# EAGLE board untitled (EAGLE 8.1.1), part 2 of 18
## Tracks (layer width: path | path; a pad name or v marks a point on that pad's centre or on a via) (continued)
S$1112
  Bottom 0: 321.52,97.17 320.59,96.24
S$1113
  Bottom 0: 320.59,96.24 320.33,96.22
S$1114
  Bottom 0: 320.33,96.22 320.22,96.19
S$1115
  Bottom 0: 320.22,96.19 319.92,96.25
S$1116
  Bottom 0: 319.92,96.25 319.57,96.22
S$1117
  Bottom 0: 319.57,96.22 319.24,96.12
S$1118
  Bottom 0: 319.24,96.12 318.94,95.93
S$1119
  Bottom 0: 318.94,95.93 318.7,95.68
S$1120
  Bottom 0: 318.7,95.68 318.53,95.37
S$1121
  Bottom 0: 318.53,95.37 318.44,95.03
S$1122
  Bottom 0: 318.44,95.03 318.44,94.68
S$1123
  Bottom 0: 318.44,94.68 318.53,94.34
S$1124
  Bottom 0: 318.53,94.34 318.7,94.03
S$1125
  Bottom 0: 318.7,94.03 318.94,93.78
S$1126
  Bottom 0: 318.94,93.78 319.24,93.59
S$1127
  Bottom 0: 319.24,93.59 319.57,93.48
S$1128
  Bottom 0: 319.57,93.48 319.92,93.46
S$1129
  Bottom 0: 319.92,93.46 320.22,93.52
S$1130
  Bottom 0: 320.22,93.52 320.33,93.48
S$1131
  Bottom 0: 320.33,93.48 320.68,93.46
S$1132
  Bottom 0: 320.68,93.46 321.03,93.52
S$1133
  Bottom 0: 321.03,93.52 321.34,93.67
S$1134
  Bottom 0: 321.34,93.67 321.61,93.9
S$1135
  Bottom 0: 321.61,93.9 321.82,94.18
S$1136
  Bottom 0: 321.82,94.18 321.94,94.51
S$1137
  Bottom 0: 321.94,94.51 321.99,94.85
S$1138
  Bottom 0: 321.99,94.85 321.94,95.2
S$1139
  Bottom 0: 321.94,95.2 321.82,95.52
S$1140
  Bottom 0: 321.82,95.52 321.61,95.81
S$1141
  Bottom 0: 321.61,95.81 321.5,95.9
S$1142
  Bottom 0: 321.5,95.9 322.27,96.68
S$1143
  Bottom 0: 322.27,96.68 322.32,96.73
S$1144
  Bottom 0: 322.32,96.73 322.35,96.79
S$1145
  Bottom 0: 322.35,96.79 322.38,96.85
S$1146
  Bottom 0: 322.38,96.85 322.4,96.92
S$1147
  Bottom 0: 322.4,96.92 322.4,96.99
S$1148
  Bottom 0: 322.4,96.99 322.4,116.07
S$1149
  Bottom 0: 322.4,116.07 323.2,116.07
S$1150
  Bottom 0: 323.2,116.07 323.28,116.08
S$1151
  Bottom 0: 323.28,116.08 323.35,116.12
S$1152
  Bottom 0: 323.35,116.12 323.41,116.18
S$1153
  Bottom 0: 323.41,116.18 323.45,116.25
S$1154
  Bottom 0: 323.45,116.25 323.46,116.33
S$1155
  Bottom 0: 323.46,116.33 323.46,144.15
S$1156
  Bottom 0: 323.46,144.15 323.45,144.22
S$1157
  Bottom 0: 323.45,144.22 323.41,144.3
S$1158
  Bottom 0: 323.41,144.3 323.35,144.35
S$1159
  Bottom 0: 323.35,144.35 323.28,144.39
S$1160
  Bottom 0: 323.28,144.39 323.2,144.4
S$1161
  Bottom 0: 323.2,144.4 322.4,144.4
S$1162
  Bottom 0: 322.4,144.4 322.4,150.63
S$1163
  Bottom 0: 322.4,150.63 322.4,150.71
S$1164
  Bottom 0: 322.4,150.71 322.38,150.77
S$1165
  Bottom 0: 322.38,150.77 322.35,150.84
S$1166
  Bottom 0: 322.35,150.84 322.32,150.9
S$1167
  Bottom 0: 322.32,150.9 322.27,150.95
S$1168
  Bottom 0: 322.27,150.95 321.84,151.38
S$1169
  Bottom 0: 321.84,151.38 321.95,151.66
S$1170
  Bottom 0: 321.95,151.66 322,152
S$1171
  Bottom 0: 322,152 321.95,152.35
S$1172
  Bottom 0: 321.95,152.35 321.82,152.67
S$1173
  Bottom 0: 321.82,152.67 321.62,152.96
S$1174
  Bottom 0: 321.62,152.96 321.35,153.18
S$1175
  Bottom 0: 321.35,153.18 321.03,153.34
S$1176
  Bottom 0: 321.03,153.34 320.69,153.39
S$1177
  Bottom 0: 320.69,153.39 320.33,153.38
S$1178
  Bottom 0: 320.33,153.38 320.23,153.34
S$1179
  Bottom 0: 320.23,153.34 319.92,153.39
S$1180
  Bottom 0: 319.92,153.39 319.68,153.38
S$1181
  Bottom 0: 319.68,153.38 322.49,156.19
S$1182
  Bottom 0: 322.49,156.19 322.53,156.25
S$1183
  Bottom 0: 322.53,156.25 322.57,156.31
S$1184
  Bottom 0: 322.57,156.31 322.6,156.37
S$1185
  Bottom 0: 322.6,156.37 322.61,156.43
S$1186
  Bottom 0: 322.61,156.43 322.62,156.5
S$1187
  Bottom 0: 322.62,156.5 322.62,171.62
S$1188
  Bottom 0: 322.62,171.62 322.61,171.69
S$1189
  Bottom 0: 322.61,171.69 322.6,171.76
S$1190
  Bottom 0: 322.6,171.76 322.57,171.82
S$1191
  Bottom 0: 322.57,171.82 322.53,171.88
S$1192
  Bottom 0: 322.53,171.88 322.49,171.94
S$1193
  Bottom 0: 322.49,171.94 318.05,176.38
S$1194
  Bottom 0: 318.05,176.38 318.06,176.42
S$1195
  Bottom 0: 318.06,176.42 318.01,176.67
S$1196
  Bottom 0: 318.01,176.67 317.88,176.89
S$1197
  Bottom 0: 317.88,176.89 317.68,177.04
S$1198
  Bottom 0: 317.68,177.04 317.43,177.1
S$1199
  Bottom 0: 317.43,177.1 317.19,177.08
S$1200
  Bottom 0: 317.19,177.08 317.06,177.02
S$1201
  Bottom 0: 317.06,177.02 317.65,177.61
S$1202
  Bottom 0: 317.65,177.61 317.9,177.54
S$1203
  Bottom 0: 317.9,177.54 318.22,177.54
S$1204
  Bottom 0: 318.22,177.54 318.53,177.63
S$1205
  Bottom 0: 318.53,177.63 318.81,177.81
S$1206
  Bottom 0: 318.81,177.81 319.02,178.05
S$1207
  Bottom 0: 319.02,178.05 319.16,178.35
S$1208
  Bottom 0: 319.16,178.35 319.2,178.67
S$1209
  Bottom 0: 319.2,178.67 319.16,178.99
S$1210
  Bottom 0: 319.16,178.99 319.02,179.29
S$1211
  Bottom 0: 319.02,179.29 318.81,179.54
S$1212
  Bottom 0: 318.81,179.54 318.53,179.72
S$1213
  Bottom 0: 318.53,179.72 318.22,179.81
S$1214
  Bottom 0: 318.22,179.81 317.9,179.81
S$1215
  Bottom 0: 317.9,179.81 317.68,179.74
S$1216
  Bottom 0: 317.68,179.74 316.95,180.46
S$1217
  Bottom 0: 316.95,180.46 316.89,180.52
S$1218
  Bottom 0: 316.89,180.52 316.81,180.57
S$1219
  Bottom 0: 316.81,180.57 316.73,180.6
S$1220
  Bottom 0: 316.73,180.6 316.64,180.62
S$1221
  Bottom 0: 316.64,180.62 316.56,180.63
S$1222
  Bottom 0: 316.56,180.63 300.39,180.63
S$1223
  Bottom 0: 300.39,180.63 300.3,180.62
S$1224
  Bottom 0: 300.3,180.62 300.21,180.6
S$1225
  Bottom 0: 300.21,180.6 300.13,180.57
S$1226
  Bottom 0: 300.13,180.57 300.06,180.52
S$1227
  Bottom 0: 300.06,180.52 299.99,180.46
S$1228
  Bottom 0: 299.99,180.46 299.29,179.77
S$1229
  Bottom 0: 299.29,179.77 299.17,179.81
S$1230
  Bottom 0: 299.17,179.81 298.84,179.81
S$1231
  Bottom 0: 298.84,179.81 298.63,179.74
S$1232
  Bottom 0: 298.63,179.74 297.9,180.46
S$1233
  Bottom 0: 297.9,180.46 297.84,180.52
S$1234
  Bottom 0: 297.84,180.52 297.76,180.57
S$1235
  Bottom 0: 297.76,180.57 297.68,180.6
S$1236
  Bottom 0: 297.68,180.6 297.6,180.62
S$1237
  Bottom 0: 297.6,180.62 297.5,180.63
S$1238
  Bottom 0: 297.5,180.63 288.83,180.63
S$1239
  Bottom 0: 288.83,180.63 288.74,180.62
S$1240
  Bottom 0: 288.74,180.62 288.66,180.6
S$1241
  Bottom 0: 288.66,180.6 288.57,180.57
S$1242
  Bottom 0: 288.57,180.57 288.5,180.52
S$1243
  Bottom 0: 288.5,180.52 288.43,180.46
S$1244
  Bottom 0: 288.43,180.46 283.51,175.54
S$1245
  Bottom 0: 283.51,175.54 283.45,175.47
S$1246
  Bottom 0: 283.45,175.47 283.4,175.4
S$1247
  Bottom 0: 283.4,175.4 283.37,175.32
S$1248
  Bottom 0: 283.37,175.32 283.35,175.23
S$1249
  Bottom 0: 283.35,175.23 283.34,175.14
S$1250
  Bottom 0: 283.34,175.14 283.34,173.77
S$1251
  Bottom 0: 283.34,173.77 283.29,173.74
S$1252
  Bottom 0: 283.29,173.74 283.22,173.68
S$1253
  Bottom 0: 283.22,173.68 281.47,171.93
S$1254
  Bottom 0: 281.47,171.93 281.41,171.86
S$1255
  Bottom 0: 281.41,171.86 281.37,171.78
S$1256
  Bottom 0: 281.37,171.78 281.33,171.7
S$1257
  Bottom 0: 281.33,171.7 281.31,171.62
S$1258
  Bottom 0: 281.31,171.62 281.31,171.53
S$1259
  Bottom 0: 281.31,171.53 281.31,167.23
S$1260
  Bottom 0: 281.31,167.23 276.44,167.23
S$1261
  Bottom 0: 276.44,167.23 276.44,169.07
S$1262
  Bottom 0: 276.44,169.07 276.44,169.16
S$1263
  Bottom 0: 276.44,169.16 276.42,169.25
S$1264
  Bottom 0: 276.42,169.25 276.38,169.33
S$1265
  Bottom 0: 276.38,169.33 276.34,169.4
S$1266
  Bottom 0: 276.34,169.4 276.28,169.47
S$1267
  Bottom 0: 276.28,169.47 266.79,178.95
S$1268
  Bottom 0: 266.79,178.95 266.78,179.01
S$1269
  Bottom 0: 266.78,179.01 266.64,179.31
S$1270
  Bottom 0: 266.64,179.31 266.43,179.55
S$1271
  Bottom 0: 266.43,179.55 266.15,179.73
S$1272
  Bottom 0: 266.15,179.73 265.85,179.82
S$1273
  Bottom 0: 265.85,179.82 265.52,179.82
S$1274
  Bottom 0: 265.52,179.82 265.21,179.73
S$1275
  Bottom 0: 265.21,179.73 264.94,179.55
S$1276
  Bottom 0: 264.94,179.55 264.72,179.31
S$1277
  Bottom 0: 264.72,179.31 264.59,179.01
S$1278
  Bottom 0: 264.59,179.01 264.54,178.69
S$1279
  Bottom 0: 264.54,178.69 264.58,178.39
S$1280
  Bottom 0: 264.58,178.39 264.29,178.09
S$1281
  Bottom 0: 264.29,178.09 264.29,179.58
S$1282
  Bottom 0: 264.29,179.58 264.28,179.65
S$1283
  Bottom 0: 264.28,179.65 264.24,179.72
S$1284
  Bottom 0: 264.24,179.72 264.18,179.78
S$1285
  Bottom 0: 264.18,179.78 264.11,179.82
S$1286
  Bottom 0: 264.11,179.82 264.03,179.83
S$1287
  Bottom 0: 264.03,179.83 262.25,179.83
S$1288
  Bottom 0: 262.25,179.83 262.18,179.82
S$1289
  Bottom 0: 262.18,179.82 262.11,179.78
S$1290
  Bottom 0: 262.11,179.78 262.05,179.72
S$1291
  Bottom 0: 262.05,179.72 262.01,179.65
S$1292
  Bottom 0: 262.01,179.65 262,179.58
S$1293
  Bottom 0: 262,179.58 262,177.87
S$1294
  Bottom 0: 262,177.87 247.42,177.87
S$1295
  Bottom 0: 247.42,177.87 245.91,179.38
S$1296
  Bottom 0: 245.91,179.38 245.84,179.45
S$1297
  Bottom 0: 245.84,179.45 245.76,179.49
S$1298
  Bottom 0: 245.76,179.49 245.68,179.53
S$1299
  Bottom 0: 245.68,179.53 245.6,179.55
S$1300
  Bottom 0: 245.6,179.55 245.51,179.55
S$1301
  Bottom 0: 245.51,179.55 237.86,179.55
S$1302
  Bottom 0: 237.86,179.55 237.58,179.73
S$1303
  Bottom 0: 237.58,179.73 237.27,179.82
S$1304
  Bottom 0: 237.27,179.82 236.94,179.82
S$1305
  Bottom 0: 236.94,179.82 236.64,179.73
S$1306
  Bottom 0: 236.64,179.73 236.36,179.55
S$1307
  Bottom 0: 236.36,179.55 236.15,179.31
S$1308
  Bottom 0: 236.15,179.31 236.01,179.01
S$1309
  Bottom 0: 236.01,179.01 235.97,178.69
S$1310
  Bottom 0: 235.97,178.69 236.01,178.37
S$1311
  Bottom 0: 236.01,178.37 236.15,178.07
S$1312
  Bottom 0: 236.15,178.07 236.36,177.82
S$1313
  Bottom 0: 236.36,177.82 236.64,177.65
S$1314
  Bottom 0: 236.64,177.65 236.94,177.56
S$1315
  Bottom 0: 236.94,177.56 237.27,177.56
S$1316
  Bottom 0: 237.27,177.56 237.58,177.65
S$1317
  Bottom 0: 237.58,177.65 237.86,177.82
S$1318
  Bottom 0: 237.86,177.82 238.07,178.07
S$1319
  Bottom 0: 238.07,178.07 238.21,178.37
S$1320
  Bottom 0: 238.21,178.37 238.21,178.41
S$1321
  Bottom 0: 238.21,178.41 243.54,178.41
S$1322
  Bottom 0: 243.54,178.41 243.45,178.35
S$1323
  Bottom 0: 243.45,178.35 243.29,178.1
S$1324
  Bottom 0: 243.29,178.1 243.19,177.81
S$1325
  Bottom 0: 243.19,177.81 243.19,177.5
S$1326
  Bottom 0: 243.19,177.5 243.21,177.48
S$1327
  Bottom 0: 243.21,177.48 237.76,172.03
S$1328
  Bottom 0: 237.76,172.03 237.72,171.98
S$1329
  Bottom 0: 237.72,171.98 237.68,171.92
S$1330
  Bottom 0: 237.68,171.92 237.65,171.86
S$1331
  Bottom 0: 237.65,171.86 237.64,171.79
S$1332
  Bottom 0: 237.64,171.79 237.63,171.72
S$1333
  Bottom 0: 237.63,171.72 237.63,169.19
S$1334
  Bottom 0: 237.63,169.19 237.64,169.12
S$1335
  Bottom 0: 237.64,169.12 237.65,169.06
S$1336
  Bottom 0: 237.65,169.06 237.68,169
S$1337
  Bottom 0: 237.68,169 237.72,168.94
S$1338
  Bottom 0: 237.72,168.94 237.76,168.88
S$1339
  Bottom 0: 237.76,168.88 244.92,161.72
S$1340
  Bottom 0: 244.92,161.72 244.92,160.78
S$1341
  Bottom 0: 244.92,160.78 244.54,160.78
S$1342
  Bottom 0: 244.54,160.78 244.54,160.91
S$1343
  Bottom 0: 244.54,160.91 244.47,161.13
S$1344
  Bottom 0: 244.47,161.13 244.31,161.29
S$1345
  Bottom 0: 244.31,161.29 244.09,161.35
S$1346
  Bottom 0: 244.09,161.35 243.75,161.35
S$1347
  Bottom 0: 243.75,161.35 242.67,162.44
S$1348
  Bottom 0: 242.67,162.44 242.72,162.57
S$1349
  Bottom 0: 242.72,162.57 242.77,162.89
S$1350
  Bottom 0: 242.77,162.89 242.72,163.22
S$1351
  Bottom 0: 242.72,163.22 242.6,163.51
S$1352
  Bottom 0: 242.6,163.51 242.39,163.77
S$1353
  Bottom 0: 242.39,163.77 242.13,163.96
S$1354
  Bottom 0: 242.13,163.96 241.82,164.06
S$1355
  Bottom 0: 241.82,164.06 241.5,164.08
S$1356
  Bottom 0: 241.5,164.08 241.18,164.02
S$1357
  Bottom 0: 241.18,164.02 240.89,163.87
S$1358
  Bottom 0: 240.89,163.87 240.66,163.65
S$1359
  Bottom 0: 240.66,163.65 240.48,163.37
S$1360
  Bottom 0: 240.48,163.37 240.4,163.06
S$1361
  Bottom 0: 240.4,163.06 240.4,162.73
S$1362
  Bottom 0: 240.4,162.73 240.48,162.42
S$1363
  Bottom 0: 240.48,162.42 240.66,162.14
S$1364
  Bottom 0: 240.66,162.14 240.89,161.92
S$1365
  Bottom 0: 240.89,161.92 241.18,161.77
S$1366
  Bottom 0: 241.18,161.77 241.5,161.71
S$1367
  Bottom 0: 241.5,161.71 241.82,161.73
S$1368
  Bottom 0: 241.82,161.73 242.04,161.8
S$1369
  Bottom 0: 242.04,161.8 243.09,160.75
S$1370
  Bottom 0: 243.09,160.75 243.06,160.73
S$1371
  Bottom 0: 243.06,160.73 243,160.68
S$1372
  Bottom 0: 243,160.68 242.96,160.6
S$1373
  Bottom 0: 242.96,160.6 242.95,160.53
S$1374
  Bottom 0: 242.95,160.53 242.95,158.75
S$1375
  Bottom 0: 242.95,158.75 242.96,158.67
S$1376
  Bottom 0: 242.96,158.67 243,158.6
S$1377
  Bottom 0: 243,158.6 243.06,158.55
S$1378
  Bottom 0: 243.06,158.55 243.13,158.51
S$1379
  Bottom 0: 243.13,158.51 243.21,158.5
S$1380
  Bottom 0: 243.21,158.5 244.98,158.5
S$1381
  Bottom 0: 244.98,158.5 245.06,158.51
S$1382
  Bottom 0: 245.06,158.51 245.13,158.55
S$1383
  Bottom 0: 245.13,158.55 245.15,158.57
S$1384
  Bottom 0: 245.15,158.57 245.67,158.05
S$1385
  Bottom 0: 245.67,158.05 237.47,158.05
S$1386
  Bottom 0: 237.47,158.05 226.48,169.04
S$1387
  Bottom 0: 226.48,169.04 226.71,169.09
S$1388
  Bottom 0: 226.71,169.09 226.97,169.25
S$1389
  Bottom 0: 226.97,169.25 227.17,169.46
S$1390
  Bottom 0: 227.17,169.46 227.31,169.74
S$1391
  Bottom 0: 227.31,169.74 227.35,170.04
S$1392
  Bottom 0: 227.35,170.04 227.31,170.34
S$1393
  Bottom 0: 227.31,170.34 227.17,170.61
S$1394
  Bottom 0: 227.17,170.61 226.97,170.83
S$1395
  Bottom 0: 226.97,170.83 226.78,170.94
S$1396
  Bottom 0: 226.78,170.94 226.78,172.36
S$1397
  Bottom 0: 226.78,172.36 226.77,172.44
S$1398
  Bottom 0: 226.77,172.44 226.76,172.5
S$1399
  Bottom 0: 226.76,172.5 226.73,172.56
S$1400
  Bottom 0: 226.73,172.56 226.69,172.62
S$1401
  Bottom 0: 226.69,172.62 226.65,172.68
S$1402
  Bottom 0: 226.65,172.68 218.94,180.39
S$1403
  Bottom 0: 218.94,180.39 218.88,180.43
S$1404
  Bottom 0: 218.88,180.43 218.82,180.47
S$1405
  Bottom 0: 218.82,180.47 218.76,180.5
S$1406
  Bottom 0: 218.76,180.5 218.69,180.51
S$1407
  Bottom 0: 218.69,180.51 218.62,180.52
S$1408
  Bottom 0: 218.62,180.52 217.66,180.52
S$1409
  Bottom 0: 217.66,180.52 217.59,180.51
S$1410
  Bottom 0: 217.59,180.51 217.53,180.5
S$1411
  Bottom 0: 217.53,180.5 217.47,180.47
S$1412
  Bottom 0: 217.47,180.47 217.4,180.43
S$1413
  Bottom 0: 217.4,180.43 217.35,180.39
S$1414
  Bottom 0: 217.35,180.39 216.64,179.68
S$1415
  Bottom 0: 216.64,179.68 216.61,179.72
S$1416
  Bottom 0: 216.61,179.72 216.56,179.78
S$1417
  Bottom 0: 216.56,179.78 216.48,179.82
S$1418
  Bottom 0: 216.48,179.82 216.41,179.83
S$1419
  Bottom 0: 216.41,179.83 214.63,179.83
S$1420
  Bottom 0: 214.63,179.83 214.55,179.82
S$1421
  Bottom 0: 214.55,179.82 214.48,179.78
S$1422
  Bottom 0: 214.48,179.78 214.43,179.72
S$1423
  Bottom 0: 214.43,179.72 214.39,179.65
S$1424
  Bottom 0: 214.39,179.65 214.38,179.58
S$1425
  Bottom 0: 214.38,179.58 214.38,177.8
S$1426
  Bottom 0: 214.38,177.8 214.39,177.72
S$1427
  Bottom 0: 214.39,177.72 214.43,177.65
S$1428
  Bottom 0: 214.43,177.65 214.48,177.6
S$1429
  Bottom 0: 214.48,177.6 214.55,177.56
S$1430
  Bottom 0: 214.55,177.56 214.63,177.55
S$1431
  Bottom 0: 214.63,177.55 215.02,177.55
S$1432
  Bottom 0: 215.02,177.55 212.37,174.9
S$1433
  Bottom 0: 212.37,174.9 212.33,174.84
S$1434
  Bottom 0: 212.33,174.84 212.29,174.78
S$1435
  Bottom 0: 212.29,174.78 212.26,174.72
S$1436
  Bottom 0: 212.26,174.72 212.25,174.66
S$1437
  Bottom 0: 212.25,174.66 212.24,174.58
S$1438
  Bottom 0: 212.24,174.58 212.24,166.18
S$1439
  Bottom 0: 212.24,166.18 212.07,166.02
S$1440
  Bottom 0: 212.07,166.02 211.9,165.75
S$1441
  Bottom 0: 211.9,165.75 211.82,165.43
S$1442
  Bottom 0: 211.82,165.43 211.82,165.1
S$1443
  Bottom 0: 211.82,165.1 211.9,164.79
S$1444
  Bottom 0: 211.9,164.79 211.98,164.67
S$1445
  Bottom 0: 211.98,164.67 209.27,167.38
S$1446
  Bottom 0: 209.27,167.38 209.22,167.42
S$1447
  Bottom 0: 209.22,167.42 209.15,167.46
S$1448
  Bottom 0: 209.15,167.46 209.09,167.48
S$1449
  Bottom 0: 209.09,167.48 209.03,167.5
S$1450
  Bottom 0: 209.03,167.5 208.96,167.5
S$1451
  Bottom 0: 208.96,167.5 205.74,167.5
S$1452
  Bottom 0: 205.74,167.5 202.79,170.45
S$1453
  Bottom 0: 202.79,170.45 202.9,170.72
S$1454
  Bottom 0: 202.9,170.72 202.95,171.07
S$1455
  Bottom 0: 202.95,171.07 202.9,171.41
S$1456
  Bottom 0: 202.9,171.41 202.77,171.74
S$1457
  Bottom 0: 202.77,171.74 202.56,172.02
S$1458
  Bottom 0: 202.56,172.02 202.3,172.25
S$1459
  Bottom 0: 202.3,172.25 201.98,172.4
S$1460
  Bottom 0: 201.98,172.4 201.63,172.46
S$1461
  Bottom 0: 201.63,172.46 201.28,172.44
S$1462
  Bottom 0: 201.28,172.44 200.96,172.33
S$1463
  Bottom 0: 200.96,172.33 200.66,172.15
S$1464
  Bottom 0: 200.66,172.15 200.42,171.89
S$1465
  Bottom 0: 200.42,171.89 200.42,171.92
S$1466
  Bottom 0: 200.42,171.92 200.66,172.16
S$1467
  Bottom 0: 200.66,172.16 200.73,172.23
S$1468
  Bottom 0: 200.73,172.23 200.77,172.3
S$1469
  Bottom 0: 200.77,172.3 200.81,172.38
S$1470
  Bottom 0: 200.81,172.38 200.83,172.47
S$1471
  Bottom 0: 200.83,172.47 200.83,172.56
S$1472
  Bottom 0: 200.83,172.56 200.83,177.43
S$1473
  Bottom 0: 200.83,177.43 200.83,177.52
S$1474
  Bottom 0: 200.83,177.52 200.81,177.61
S$1475
  Bottom 0: 200.81,177.61 200.77,177.69
S$1476
  Bottom 0: 200.77,177.69 200.73,177.76
S$1477
  Bottom 0: 200.73,177.76 200.66,177.83
S$1478
  Bottom 0: 200.66,177.83 200.11,178.39
S$1479
  Bottom 0: 200.11,178.39 200.15,178.69
S$1480
  Bottom 0: 200.15,178.69 200.11,179.01
S$1481
  Bottom 0: 200.11,179.01 199.97,179.31
S$1482
  Bottom 0: 199.97,179.31 199.76,179.55
S$1483
  Bottom 0: 199.76,179.55 199.48,179.73
S$1484
  Bottom 0: 199.48,179.73 199.17,179.82
S$1485
  Bottom 0: 199.17,179.82 198.84,179.82
S$1486
  Bottom 0: 198.84,179.82 198.54,179.73
S$1487
  Bottom 0: 198.54,179.73 198.26,179.55
S$1488
  Bottom 0: 198.26,179.55 198.17,179.44
S$1489
  Bottom 0: 198.17,179.44 198.17,179.84
S$1490
  Bottom 0: 198.17,179.84 198.16,179.91
S$1491
  Bottom 0: 198.16,179.91 198.14,179.97
S$1492
  Bottom 0: 198.14,179.97 198.12,180.03
S$1493
  Bottom 0: 198.12,180.03 198.08,180.1
S$1494
  Bottom 0: 198.08,180.1 198.04,180.15
S$1495
  Bottom 0: 198.04,180.15 197.93,180.26
S$1496
  Bottom 0: 197.93,180.26 197.87,180.3
S$1497
  Bottom 0: 197.87,180.3 197.81,180.34
S$1498
  Bottom 0: 197.81,180.34 197.75,180.37
S$1499
  Bottom 0: 197.75,180.37 197.68,180.39
S$1500
  Bottom 0: 197.68,180.39 197.61,180.39
S$1501
  Bottom 0: 197.61,180.39 195.35,180.39
S$1502
  Bottom 0: 195.35,180.39 195.28,180.39
S$1503
  Bottom 0: 195.28,180.39 195.21,180.37
S$1504
  Bottom 0: 195.21,180.37 195.15,180.34
S$1505
  Bottom 0: 195.15,180.34 195.03,180.26
S$1506
  Bottom 0: 195.03,180.26 186.29,171.51
S$1507
  Bottom 0: 186.29,171.51 183.81,171.51
S$1508
  Bottom 0: 183.81,171.51 183.72,171.74
S$1509
  Bottom 0: 183.72,171.74 183.51,172.02
S$1510
  Bottom 0: 183.51,172.02 183.25,172.25
S$1511
  Bottom 0: 183.25,172.25 182.93,172.4
S$1512
  Bottom 0: 182.93,172.4 182.58,172.46
S$1513
  Bottom 0: 182.58,172.46 182.24,172.44
S$1514
  Bottom 0: 182.24,172.44 181.91,172.33
S$1515
  Bottom 0: 181.91,172.33 181.61,172.15
S$1516
  Bottom 0: 181.61,172.15 181.37,171.89
S$1517
  Bottom 0: 181.37,171.89 181.2,171.58
S$1518
  Bottom 0: 181.2,171.58 181.11,171.24
S$1519
  Bottom 0: 181.11,171.24 181.11,170.9
S$1520
  Bottom 0: 181.11,170.9 181.2,170.56
S$1521
  Bottom 0: 181.2,170.56 181.37,170.25
S$1522
  Bottom 0: 181.37,170.25 181.61,169.99
S$1523
  Bottom 0: 181.61,169.99 181.91,169.8
S$1524
  Bottom 0: 181.91,169.8 182.24,169.7
S$1525
  Bottom 0: 182.24,169.7 182.58,169.68
S$1526
  Bottom 0: 182.58,169.68 182.93,169.74
S$1527
  Bottom 0: 182.93,169.74 183.25,169.89
S$1528
  Bottom 0: 183.25,169.89 183.51,170.11
S$1529
  Bottom 0: 183.51,170.11 183.72,170.4
S$1530
  Bottom 0: 183.72,170.4 183.81,170.63
S$1531
  Bottom 0: 183.81,170.63 186.23,170.63
S$1532
  Bottom 0: 186.23,170.63 186.13,170.48
S$1533
  Bottom 0: 186.13,170.48 186.04,170.19
S$1534
  Bottom 0: 186.04,170.19 186.04,169.88
S$1535
  Bottom 0: 186.04,169.88 186.13,169.6
S$1536
  Bottom 0: 186.13,169.6 186.3,169.35
S$1537
  Bottom 0: 186.3,169.35 186.54,169.16
S$1538
  Bottom 0: 186.54,169.16 186.82,169.05
S$1539
  Bottom 0: 186.82,169.05 187.12,169.03
S$1540
  Bottom 0: 187.12,169.03 187.41,169.09
S$1541
  Bottom 0: 187.41,169.09 187.68,169.25
S$1542
  Bottom 0: 187.68,169.25 187.88,169.46
S$1543
  Bottom 0: 187.88,169.46 188.02,169.74
S$1544
  Bottom 0: 188.02,169.74 188.06,170.04
S$1545
  Bottom 0: 188.06,170.04 188.02,170.34
S$1546
  Bottom 0: 188.02,170.34 187.88,170.61
S$1547
  Bottom 0: 187.88,170.61 187.68,170.83
S$1548
  Bottom 0: 187.68,170.83 187.41,170.98
S$1549
  Bottom 0: 187.41,170.98 187.12,171.05
S$1550
  Bottom 0: 187.12,171.05 187.08,171.04
S$1551
  Bottom 0: 187.08,171.04 195.33,179.29
S$1552
  Bottom 0: 195.33,179.29 195.33,177.8
S$1553
  Bottom 0: 195.33,177.8 195.34,177.72
S$1554
  Bottom 0: 195.34,177.72 195.38,177.65
S$1555
  Bottom 0: 195.38,177.65 195.43,177.6
S$1556
  Bottom 0: 195.43,177.6 195.5,177.56
S$1557
  Bottom 0: 195.5,177.56 195.58,177.55
S$1558
  Bottom 0: 195.58,177.55 195.97,177.55
S$1559
  Bottom 0: 195.97,177.55 193.24,174.82
S$1560
  Bottom 0: 193.24,174.82 193.19,174.77
S$1561
  Bottom 0: 193.19,174.77 193.16,174.71
S$1562
  Bottom 0: 193.16,174.71 193.13,174.65
S$1563
  Bottom 0: 193.13,174.65 193.12,174.58
S$1564
  Bottom 0: 193.12,174.58 193.11,174.51
S$1565
  Bottom 0: 193.11,174.51 193.11,166.1
S$1566
  Bottom 0: 193.11,166.1 193.03,166.02
S$1567
  Bottom 0: 193.03,166.02 192.85,165.75
S$1568
  Bottom 0: 192.85,165.75 192.77,165.43
S$1569
  Bottom 0: 192.77,165.43 192.77,165.1
S$1570
  Bottom 0: 192.77,165.1 192.85,164.79
S$1571
  Bottom 0: 192.85,164.79 192.93,164.67
S$1572
  Bottom 0: 192.93,164.67 190.66,166.93
S$1573
  Bottom 0: 190.66,166.93 190.61,166.97
S$1574
  Bottom 0: 190.61,166.97 190.55,167.01
S$1575
  Bottom 0: 190.55,167.01 190.49,167.03
S$1576
  Bottom 0: 190.49,167.03 190.42,167.05
S$1577
  Bottom 0: 190.42,167.05 190.35,167.06
S$1578
  Bottom 0: 190.35,167.06 180.77,167.06
S$1579
  Bottom 0: 180.77,167.06 180.7,167.05
S$1580
  Bottom 0: 180.7,167.05 180.63,167.03
S$1581
  Bottom 0: 180.63,167.03 180.57,167.01
S$1582
  Bottom 0: 180.57,167.01 180.51,166.97
S$1583
  Bottom 0: 180.51,166.97 180.46,166.93
S$1584
  Bottom 0: 180.46,166.93 177.93,164.4
S$1585
  Bottom 0: 177.93,164.4 175.72,164.4
S$1586
  Bottom 0: 175.72,164.4 175.92,164.65
S$1587
  Bottom 0: 175.92,164.65 176.04,164.95
S$1588
  Bottom 0: 176.04,164.95 176.09,165.27
S$1589
  Bottom 0: 176.09,165.27 176.04,165.59
S$1590
  Bottom 0: 176.04,165.59 175.92,165.89
S$1591
  Bottom 0: 175.92,165.89 175.71,166.14
S$1592
  Bottom 0: 175.71,166.14 175.45,166.33
S$1593
  Bottom 0: 175.45,166.33 175.14,166.44
S$1594
  Bottom 0: 175.14,166.44 175.06,166.44
S$1595
  Bottom 0: 175.06,166.44 175.06,167.67
S$1596
  Bottom 0: 175.06,167.67 175.26,167.45
S$1597
  Bottom 0: 175.26,167.45 175.56,167.26
S$1598
  Bottom 0: 175.56,167.26 175.88,167.16
S$1599
  Bottom 0: 175.88,167.16 176.23,167.14
S$1600
  Bottom 0: 176.23,167.14 176.58,167.2
S$1601
  Bottom 0: 176.58,167.2 176.9,167.35
S$1602
  Bottom 0: 176.9,167.35 177.16,167.57
S$1603
  Bottom 0: 177.16,167.57 177.37,167.86
S$1604
  Bottom 0: 177.37,167.86 177.47,168.09
S$1605
  Bottom 0: 177.47,168.09 187.91,168.09
S$1606
  Bottom 0: 187.91,168.09 187.98,168.09
S$1607
  Bottom 0: 187.98,168.09 188.05,168.11
S$1608
  Bottom 0: 188.05,168.11 188.11,168.13
S$1609
  Bottom 0: 188.11,168.13 188.17,168.17
S$1610
  Bottom 0: 188.17,168.17 188.23,168.21
S$1611
  Bottom 0: 188.23,168.21 189.1,169.08
S$1612
  Bottom 0: 189.1,169.08 189.19,169.05
S$1613
  Bottom 0: 189.19,169.05 189.5,169.03
S$1614
  Bottom 0: 189.5,169.03 189.79,169.09
S$1615
  Bottom 0: 189.79,169.09 190.06,169.25
S$1616
  Bottom 0: 190.06,169.25 190.26,169.46
S$1617
  Bottom 0: 190.26,169.46 190.39,169.74
S$1618
  Bottom 0: 190.39,169.74 190.44,170.04
S$1619
  Bottom 0: 190.44,170.04 190.39,170.34
S$1620
  Bottom 0: 190.39,170.34 190.26,170.61
S$1621
  Bottom 0: 190.26,170.61 190.06,170.83
S$1622
  Bottom 0: 190.06,170.83 189.79,170.98
S$1623
  Bottom 0: 189.79,170.98 189.5,171.05
S$1624
  Bottom 0: 189.5,171.05 189.19,171.03
S$1625
  Bottom 0: 189.19,171.03 188.91,170.92
S$1626
  Bottom 0: 188.91,170.92 188.68,170.73
S$1627
  Bottom 0: 188.68,170.73 188.51,170.48
S$1628
  Bottom 0: 188.51,170.48 188.42,170.19
S$1629
  Bottom 0: 188.42,170.19 188.42,169.88
S$1630
  Bottom 0: 188.42,169.88 188.47,169.72
S$1631
  Bottom 0: 188.47,169.72 187.73,168.97
S$1632
  Bottom 0: 187.73,168.97 177.47,168.97
S$1633
  Bottom 0: 177.47,168.97 177.37,169.2
S$1634
  Bottom 0: 177.37,169.2 177.16,169.48
S$1635
  Bottom 0: 177.16,169.48 176.9,169.71
S$1636
  Bottom 0: 176.9,169.71 176.58,169.86
S$1637
  Bottom 0: 176.58,169.86 176.23,169.92
S$1638
  Bottom 0: 176.23,169.92 175.88,169.9
S$1639
  Bottom 0: 175.88,169.9 175.56,169.79
S$1640
  Bottom 0: 175.56,169.79 175.26,169.61
S$1641
  Bottom 0: 175.26,169.61 175.06,169.39
S$1642
  Bottom 0: 175.06,169.39 175.06,174.44
S$1643
  Bottom 0: 175.06,174.44 177.73,177.1
S$1644
  Bottom 0: 177.73,177.1 177.76,177.16
S$1645
  Bottom 0: 177.76,177.16 177.8,177.2
S$1646
  Bottom 0: 177.8,177.2 177.81,177.25
S$1647
  Bottom 0: 177.81,177.25 177.85,177.3
S$1648
  Bottom 0: 177.85,177.3 177.85,177.36
S$1649
  Bottom 0: 177.85,177.36 177.86,177.42
S$1650
  Bottom 0: 177.86,177.42 177.86,177.55
S$1651
  Bottom 0: 177.86,177.55 178.31,177.55
S$1652
  Bottom 0: 178.31,177.55 178.38,177.56
S$1653
  Bottom 0: 178.38,177.56 178.46,177.6
S$1654
  Bottom 0: 178.46,177.6 178.51,177.65
S$1655
  Bottom 0: 178.51,177.65 178.55,177.72
S$1656
  Bottom 0: 178.55,177.72 178.56,177.8
S$1657
  Bottom 0: 178.56,177.8 178.56,179.51
S$1658
  Bottom 0: 178.56,179.51 179.17,179.51
S$1659
  Bottom 0: 179.17,179.51 179,179.31
S$1660
  Bottom 0: 179,179.31 178.86,179.01
S$1661
  Bottom 0: 178.86,179.01 178.82,178.69
S$1662
  Bottom 0: 178.82,178.69 178.86,178.37
S$1663
  Bottom 0: 178.86,178.37 179,178.07
S$1664
  Bottom 0: 179,178.07 179.21,177.82
S$1665
  Bottom 0: 179.21,177.82 179.49,177.65
S$1666
  Bottom 0: 179.49,177.65 179.79,177.56
S$1667
  Bottom 0: 179.79,177.56 180.12,177.56
S$1668
  Bottom 0: 180.12,177.56 180.43,177.65
S$1669
  Bottom 0: 180.43,177.65 180.71,177.82
S$1670
  Bottom 0: 180.71,177.82 180.92,178.07
S$1671
  Bottom 0: 180.92,178.07 181.06,178.37
S$1672
  Bottom 0: 181.06,178.37 181.1,178.69
S$1673
  Bottom 0: 181.1,178.69 181.06,179.01
S$1674
  Bottom 0: 181.06,179.01 180.92,179.31
S$1675
  Bottom 0: 180.92,179.31 180.74,179.51
S$1676
  Bottom 0: 180.74,179.51 186.94,179.51
S$1677
  Bottom 0: 186.94,179.51 188.47,177.98
S$1678
  Bottom 0: 188.47,177.98 188.42,177.81
S$1679
  Bottom 0: 188.42,177.81 188.42,177.5
S$1680
  Bottom 0: 188.42,177.5 188.51,177.22
S$1681
  Bottom 0: 188.51,177.22 188.68,176.97
S$1682
  Bottom 0: 188.68,176.97 188.91,176.78
S$1683
  Bottom 0: 188.91,176.78 189.19,176.67
S$1684
  Bottom 0: 189.19,176.67 189.5,176.65
S$1685
  Bottom 0: 189.5,176.65 189.79,176.71
S$1686
  Bottom 0: 189.79,176.71 190.06,176.87
S$1687
  Bottom 0: 190.06,176.87 190.26,177.08
S$1688
  Bottom 0: 190.26,177.08 190.39,177.36
S$1689
  Bottom 0: 190.39,177.36 190.44,177.66
S$1690
  Bottom 0: 190.44,177.66 190.39,177.96
S$1691
  Bottom 0: 190.39,177.96 190.26,178.23
S$1692
  Bottom 0: 190.26,178.23 190.06,178.45
S$1693
  Bottom 0: 190.06,178.45 189.79,178.6
S$1694
  Bottom 0: 189.79,178.6 189.5,178.67
S$1695
  Bottom 0: 189.5,178.67 189.19,178.65
S$1696
  Bottom 0: 189.19,178.65 189.1,178.61
S$1697
  Bottom 0: 189.1,178.61 187.45,180.26
S$1698
  Bottom 0: 187.45,180.26 187.39,180.3
S$1699
  Bottom 0: 187.39,180.3 187.33,180.34
S$1700
  Bottom 0: 187.33,180.34 187.27,180.37
S$1701
  Bottom 0: 187.27,180.37 187.2,180.39
S$1702
  Bottom 0: 187.2,180.39 187.13,180.39
S$1703
  Bottom 0: 187.13,180.39 80.72,180.39
S$1704
  Bottom 0: 80.72,180.39 80.65,180.39
S$1705
  Bottom 0: 80.65,180.39 80.58,180.37
S$1706
  Bottom 0: 80.58,180.37 80.52,180.34
S$1707
  Bottom 0: 80.52,180.34 80.46,180.3
S$1708
  Bottom 0: 80.46,180.3 80.4,180.26
S$1709
  Bottom 0: 80.4,180.26 58.88,158.74
S$1710
  Bottom 0: 58.88,158.74 56.83,158.74
S$1711
  Bottom 0: 56.83,158.74 56.88,158.78
S$1712
  Bottom 0: 56.88,158.78 57.09,159.02
S$1713
  Bottom 0: 57.09,159.02 57.23,159.32
S$1714
  Bottom 0: 57.23,159.32 57.28,159.64
S$1715
  Bottom 0: 57.28,159.64 57.23,159.96
S$1716
  Bottom 0: 57.23,159.96 57.09,160.26
S$1717
  Bottom 0: 57.09,160.26 56.88,160.5
S$1718
  Bottom 0: 56.88,160.5 56.61,160.68
S$1719
  Bottom 0: 56.61,160.68 56.3,160.77
S$1720
  Bottom 0: 56.3,160.77 55.97,160.77
S$1721
  Bottom 0: 55.97,160.77 55.66,160.68
S$1722
  Bottom 0: 55.66,160.68 55.38,160.5
S$1723
  Bottom 0: 55.38,160.5 55.17,160.26
S$1724
  Bottom 0: 55.17,160.26 55.03,159.96
S$1725
  Bottom 0: 55.03,159.96 54.99,159.64
S$1726
  Bottom 0: 54.99,159.64 55.03,159.32
S$1727
  Bottom 0: 55.03,159.32 55.17,159.02
S$1728
  Bottom 0: 55.17,159.02 55.38,158.78
S$1729
  Bottom 0: 55.38,158.78 55.44,158.74
S$1730
  Bottom 0: 55.44,158.74 54.74,158.74
S$1731
  Bottom 0: 54.74,158.74 54.74,160.53
S$1732
  Bottom 0: 54.74,160.53 54.73,160.6
S$1733
  Bottom 0: 54.73,160.6 54.68,160.68
S$1734
  Bottom 0: 54.68,160.68 54.63,160.73
S$1735
  Bottom 0: 54.63,160.73 54.56,160.77
S$1736
  Bottom 0: 54.56,160.77 54.48,160.78
S$1737
  Bottom 0: 54.48,160.78 54.04,160.78
S$1738
  Bottom 0: 54.04,160.78 54.04,160.91
S$1739
  Bottom 0: 54.04,160.91 53.98,161.13
S$1740
  Bottom 0: 53.98,161.13 53.81,161.29
S$1741
  Bottom 0: 53.81,161.29 53.59,161.35
S$1742
  Bottom 0: 53.59,161.35 53.23,161.35
S$1743
  Bottom 0: 53.23,161.35 52.14,162.44
S$1744
  Bottom 0: 52.14,162.44 52.2,162.58
S$1745
  Bottom 0: 52.2,162.58 52.25,162.9
S$1746
  Bottom 0: 52.25,162.9 52.2,163.22
S$1747
  Bottom 0: 52.2,163.22 52.08,163.52
S$1748
  Bottom 0: 52.08,163.52 51.87,163.77
S$1749
  Bottom 0: 51.87,163.77 51.6,163.96
S$1750
  Bottom 0: 51.6,163.96 51.3,164.07
S$1751
  Bottom 0: 51.3,164.07 50.98,164.09
S$1752
  Bottom 0: 50.98,164.09 50.66,164.02
S$1753
  Bottom 0: 50.66,164.02 50.37,163.88
S$1754
  Bottom 0: 50.37,163.88 50.13,163.65
S$1755
  Bottom 0: 50.13,163.65 49.96,163.38
S$1756
  Bottom 0: 49.96,163.38 49.88,163.06
S$1757
  Bottom 0: 49.88,163.06 49.88,162.74
S$1758
  Bottom 0: 49.88,162.74 49.96,162.42
S$1759
  Bottom 0: 49.96,162.42 50.13,162.15
S$1760
  Bottom 0: 50.13,162.15 50.37,161.93
S$1761
  Bottom 0: 50.37,161.93 50.66,161.78
S$1762
  Bottom 0: 50.66,161.78 50.98,161.71
S$1763
  Bottom 0: 50.98,161.71 51.3,161.73
S$1764
  Bottom 0: 51.3,161.73 51.52,161.81
S$1765
  Bottom 0: 51.52,161.81 52.58,160.75
S$1766
  Bottom 0: 52.58,160.75 52.55,160.73
S$1767
  Bottom 0: 52.55,160.73 52.5,160.68
S$1768
  Bottom 0: 52.5,160.68 52.46,160.6
S$1769
  Bottom 0: 52.46,160.6 52.45,160.53
S$1770
  Bottom 0: 52.45,160.53 52.45,159.09
S$1771
  Bottom 0: 52.45,159.09 51.49,160.05
S$1772
  Bottom 0: 51.49,160.05 51.44,160.09
S$1773
  Bottom 0: 51.44,160.09 51.37,160.13
S$1774
  Bottom 0: 51.37,160.13 51.31,160.16
S$1775
  Bottom 0: 51.31,160.16 51.25,160.17
S$1776
  Bottom 0: 51.25,160.17 51.18,160.18
S$1777
  Bottom 0: 51.18,160.18 39.13,160.18
S$1778
  Bottom 0: 39.13,160.18 39.06,160.17
S$1779
  Bottom 0: 39.06,160.17 38.99,160.16
S$1780
  Bottom 0: 38.99,160.16 38.93,160.13
S$1781
  Bottom 0: 38.93,160.13 38.87,160.09
S$1782
  Bottom 0: 38.87,160.09 38.82,160.05
S$1783
  Bottom 0: 38.82,160.05 38.2,159.43
S$1784
  Bottom 0: 38.2,159.43 38.23,159.64
S$1785
  Bottom 0: 38.23,159.64 38.18,159.96
S$1786
  Bottom 0: 38.18,159.96 38.04,160.26
S$1787
  Bottom 0: 38.04,160.26 37.83,160.5
S$1788
  Bottom 0: 37.83,160.5 37.56,160.68
S$1789
  Bottom 0: 37.56,160.68 37.24,160.77
S$1790
  Bottom 0: 37.24,160.77 36.92,160.77
S$1791
  Bottom 0: 36.92,160.77 36.61,160.68
S$1792
  Bottom 0: 36.61,160.68 36.34,160.5
S$1793
  Bottom 0: 36.34,160.5 36.12,160.26
S$1794
  Bottom 0: 36.12,160.26 35.98,159.96
S$1795
  Bottom 0: 35.98,159.96 35.94,159.64
S$1796
  Bottom 0: 35.94,159.64 35.98,159.32
S$1797
  Bottom 0: 35.98,159.32 36.12,159.02
S$1798
  Bottom 0: 36.12,159.02 36.34,158.78
S$1799
  Bottom 0: 36.34,158.78 36.44,158.71
S$1800
  Bottom 0: 36.44,158.71 35.68,158.71
S$1801
  Bottom 0: 35.68,158.71 35.69,158.75
S$1802
  Bottom 0: 35.69,158.75 35.69,160.53
S$1803
  Bottom 0: 35.69,160.53 35.68,160.6
S$1804
  Bottom 0: 35.68,160.6 35.63,160.68
S$1805
  Bottom 0: 35.63,160.68 35.58,160.73
S$1806
  Bottom 0: 35.58,160.73 35.51,160.77
S$1807
  Bottom 0: 35.51,160.77 35.43,160.78
S$1808
  Bottom 0: 35.43,160.78 34.99,160.78
S$1809
  Bottom 0: 34.99,160.78 34.99,160.91
S$1810
  Bottom 0: 34.99,160.91 34.92,161.13
S$1811
  Bottom 0: 34.92,161.13 34.76,161.29
S$1812
  Bottom 0: 34.76,161.29 34.54,161.35
S$1813
  Bottom 0: 34.54,161.35 34.18,161.35
S$1814
  Bottom 0: 34.18,161.35 33.1,162.44
S$1815
  Bottom 0: 33.1,162.44 33.16,162.57
S$1816
  Bottom 0: 33.16,162.57 33.2,162.89
S$1817
  Bottom 0: 33.2,162.89 33.16,163.22
S$1818
  Bottom 0: 33.16,163.22 33.03,163.51
S$1819
  Bottom 0: 33.03,163.51 32.82,163.77
S$1820
  Bottom 0: 32.82,163.77 32.56,163.96
S$1821
  Bottom 0: 32.56,163.96 32.25,164.06
S$1822
  Bottom 0: 32.25,164.06 31.93,164.08
S$1823
  Bottom 0: 31.93,164.08 31.61,164.02
S$1824
  Bottom 0: 31.61,164.02 31.32,163.87
S$1825
  Bottom 0: 31.32,163.87 31.09,163.65
S$1826
  Bottom 0: 31.09,163.65 30.91,163.37
S$1827
  Bottom 0: 30.91,163.37 30.82,163.06
S$1828
  Bottom 0: 30.82,163.06 30.82,162.73
S$1829
  Bottom 0: 30.82,162.73 30.91,162.42
S$1830
  Bottom 0: 30.91,162.42 31.09,162.14
S$1831
  Bottom 0: 31.09,162.14 31.32,161.92
S$1832
  Bottom 0: 31.32,161.92 31.61,161.77
S$1833
  Bottom 0: 31.61,161.77 31.93,161.71
S$1834
  Bottom 0: 31.93,161.71 32.25,161.73
S$1835
  Bottom 0: 32.25,161.73 32.47,161.8
S$1836
  Bottom 0: 32.47,161.8 33.53,160.75
S$1837
  Bottom 0: 33.53,160.75 33.51,160.73
S$1838
  Bottom 0: 33.51,160.73 33.45,160.68
S$1839
  Bottom 0: 33.45,160.68 33.41,160.6
S$1840
  Bottom 0: 33.41,160.6 33.4,160.53
S$1841
  Bottom 0: 33.4,160.53 33.4,158.75
S$1842
  Bottom 0: 33.4,158.75 33.4,158.71
S$1843
  Bottom 0: 33.4,158.71 27.29,158.71
S$1844
  Bottom 0: 27.29,158.71 27.26,158.91
S$1845
  Bottom 0: 27.26,158.91 27.13,159.18
S$1846
  Bottom 0: 27.13,159.18 26.92,159.4
S$1847
  Bottom 0: 26.92,159.4 26.66,159.55
S$1848
  Bottom 0: 26.66,159.55 26.36,159.62
S$1849
  Bottom 0: 26.36,159.62 26.06,159.6
S$1850
  Bottom 0: 26.06,159.6 25.78,159.49
S$1851
  Bottom 0: 25.78,159.49 25.54,159.3
S$1852
  Bottom 0: 25.54,159.3 25.37,159.05
S$1853
  Bottom 0: 25.37,159.05 25.28,158.76
S$1854
  Bottom 0: 25.28,158.76 25.28,158.49
S$1855
  Bottom 0: 25.28,158.49 25.26,158.51
S$1856
  Bottom 0: 25.26,158.51 25.26,165.09
S$1857
  Bottom 0: 25.26,165.09 25.26,165.16
S$1858
  Bottom 0: 25.26,165.16 25.24,165.23
S$1859
  Bottom 0: 25.24,165.23 25.21,165.29
S$1860
  Bottom 0: 25.21,165.29 25.18,165.35
S$1861
  Bottom 0: 25.18,165.35 25.13,165.41
S$1862
  Bottom 0: 25.13,165.41 23.33,167.21
S$1863
  Bottom 0: 23.33,167.21 23.48,167.16
S$1864
  Bottom 0: 23.48,167.16 23.83,167.14
S$1865
  Bottom 0: 23.83,167.14 24.18,167.2
S$1866
  Bottom 0: 24.18,167.2 24.5,167.35
S$1867
  Bottom 0: 24.5,167.35 24.77,167.57
S$1868
  Bottom 0: 24.77,167.57 24.97,167.86
S$1869
  Bottom 0: 24.97,167.86 25.07,168.09
S$1870
  Bottom 0: 25.07,168.09 31.16,168.09
S$1871
  Bottom 0: 31.16,168.09 31.24,168.09
S$1872
  Bottom 0: 31.24,168.09 31.3,168.11
S$1873
  Bottom 0: 31.3,168.11 31.36,168.13
S$1874
  Bottom 0: 31.36,168.13 31.43,168.17
S$1875
  Bottom 0: 31.43,168.17 31.48,168.21
S$1876
  Bottom 0: 31.48,168.21 33.7,170.43
S$1877
  Bottom 0: 33.7,170.43 33.62,170.19
S$1878
  Bottom 0: 33.62,170.19 33.62,169.88
S$1879
  Bottom 0: 33.62,169.88 33.72,169.6
S$1880
  Bottom 0: 33.72,169.6 33.88,169.35
S$1881
  Bottom 0: 33.88,169.35 34.12,169.16
S$1882
  Bottom 0: 34.12,169.16 34.4,169.05
S$1883
  Bottom 0: 34.4,169.05 34.7,169.03
S$1884
  Bottom 0: 34.7,169.03 35,169.09
S$1885
  Bottom 0: 35,169.09 35.26,169.25
S$1886
  Bottom 0: 35.26,169.25 35.47,169.46
S$1887
  Bottom 0: 35.47,169.46 35.6,169.74
S$1888
  Bottom 0: 35.6,169.74 35.65,170.04
S$1889
  Bottom 0: 35.65,170.04 35.6,170.34
S$1890
  Bottom 0: 35.6,170.34 35.47,170.61
S$1891
  Bottom 0: 35.47,170.61 35.35,170.74
S$1892
  Bottom 0: 35.35,170.74 35.67,170.74
S$1893
  Bottom 0: 35.67,170.74 36.06,170.36
S$1894
  Bottom 0: 36.06,170.36 36,170.19
S$1895
  Bottom 0: 36,170.19 36,169.88
S$1896
  Bottom 0: 36,169.88 36.09,169.6
S$1897
  Bottom 0: 36.09,169.6 36.26,169.35
S$1898
  Bottom 0: 36.26,169.35 36.5,169.16
S$1899
  Bottom 0: 36.5,169.16 36.78,169.05
S$1900
  Bottom 0: 36.78,169.05 37.08,169.03
S$1901
  Bottom 0: 37.08,169.03 37.38,169.09
S$1902
  Bottom 0: 37.38,169.09 37.64,169.25
S$1903
  Bottom 0: 37.64,169.25 37.85,169.46
S$1904
  Bottom 0: 37.85,169.46 37.98,169.74
S$1905
  Bottom 0: 37.98,169.74 38.02,170.04
S$1906
  Bottom 0: 38.02,170.04 37.98,170.34
S$1907
  Bottom 0: 37.98,170.34 37.85,170.61
S$1908
  Bottom 0: 37.85,170.61 37.64,170.83
S$1909
  Bottom 0: 37.64,170.83 37.38,170.98
S$1910
  Bottom 0: 37.38,170.98 37.08,171.05
S$1911
  Bottom 0: 37.08,171.05 36.78,171.03
S$1912
  Bottom 0: 36.78,171.03 36.67,170.99
S$1913
  Bottom 0: 36.67,170.99 36.16,171.5
S$1914
  Bottom 0: 36.16,171.5 36.11,171.54
S$1915
  Bottom 0: 36.11,171.54 36.05,171.58
S$1916
  Bottom 0: 36.05,171.58 35.99,171.61
S$1917
  Bottom 0: 35.99,171.61 35.93,171.62
S$1918
  Bottom 0: 35.93,171.62 35.85,171.63
S$1919
  Bottom 0: 35.85,171.63 33.82,171.63
S$1920
  Bottom 0: 33.82,171.63 33.75,171.62
S$1921
  Bottom 0: 33.75,171.62 33.69,171.61
S$1922
  Bottom 0: 33.69,171.61 33.62,171.58
S$1923
  Bottom 0: 33.62,171.58 33.56,171.54
S$1924
  Bottom 0: 33.56,171.54 33.51,171.5
S$1925
  Bottom 0: 33.51,171.5 30.98,168.97
S$1926
  Bottom 0: 30.98,168.97 25.07,168.97
S$1927
  Bottom 0: 25.07,168.97 24.97,169.2
S$1928
  Bottom 0: 24.97,169.2 24.77,169.48
S$1929
  Bottom 0: 24.77,169.48 24.5,169.71
S$1930
  Bottom 0: 24.5,169.71 24.18,169.86
S$1931
  Bottom 0: 24.18,169.86 23.83,169.92
S$1932
  Bottom 0: 23.83,169.92 23.54,169.91
S$1933
  Bottom 0: 23.54,169.91 24.26,170.63
S$1934
  Bottom 0: 24.26,170.63 28.78,170.63
S$1935
  Bottom 0: 28.78,170.63 28.8,170.56
S$1936
  Bottom 0: 28.8,170.56 28.97,170.25
S$1937
  Bottom 0: 28.97,170.25 29.21,169.99
S$1938
  Bottom 0: 29.21,169.99 29.5,169.8
S$1939
  Bottom 0: 29.5,169.8 29.83,169.7
S$1940
  Bottom 0: 29.83,169.7 30.18,169.68
S$1941
  Bottom 0: 30.18,169.68 30.53,169.74
S$1942
  Bottom 0: 30.53,169.74 30.85,169.89
S$1943
  Bottom 0: 30.85,169.89 31.11,170.11
S$1944
  Bottom 0: 31.11,170.11 31.32,170.4
S$1945
  Bottom 0: 31.32,170.4 31.45,170.72
S$1946
  Bottom 0: 31.45,170.72 31.5,171.07
S$1947
  Bottom 0: 31.5,171.07 31.45,171.41
S$1948
  Bottom 0: 31.45,171.41 31.32,171.74
S$1949
  Bottom 0: 31.32,171.74 31.11,172.02
S$1950
  Bottom 0: 31.11,172.02 30.85,172.25
S$1951
  Bottom 0: 30.85,172.25 30.53,172.4
S$1952
  Bottom 0: 30.53,172.4 30.18,172.46
S$1953
  Bottom 0: 30.18,172.46 29.83,172.44
S$1954
  Bottom 0: 29.83,172.44 29.5,172.33
S$1955
  Bottom 0: 29.5,172.33 29.21,172.15
S$1956
  Bottom 0: 29.21,172.15 28.97,171.89
S$1957
  Bottom 0: 28.97,171.89 28.8,171.58
S$1958
  Bottom 0: 28.8,171.58 28.78,171.51
S$1959
  Bottom 0: 28.78,171.51 27.19,171.51
S$1960
  Bottom 0: 27.19,171.51 27.56,171.71
S$1961
  Bottom 0: 27.56,171.71 27.9,171.99
S$1962
  Bottom 0: 27.9,171.99 28.19,172.34
S$1963
  Bottom 0: 28.19,172.34 28.4,172.74
S$1964
  Bottom 0: 28.4,172.74 28.53,173.16
S$1965
  Bottom 0: 28.53,173.16 28.57,173.61
S$1966
  Bottom 0: 28.57,173.61 28.53,174.06
S$1967
  Bottom 0: 28.53,174.06 28.4,174.48
S$1968
  Bottom 0: 28.4,174.48 28.19,174.88
S$1969
  Bottom 0: 28.19,174.88 27.9,175.22
S$1970
  Bottom 0: 27.9,175.22 27.56,175.51
S$1971
  Bottom 0: 27.56,175.51 27.16,175.72
S$1972
  Bottom 0: 27.16,175.72 26.74,175.85
S$1973
  Bottom 0: 26.74,175.85 26.29,175.9
S$1974
  Bottom 0: 26.29,175.9 25.84,175.85
S$1975
  Bottom 0: 25.84,175.85 25.41,175.72
S$1976
  Bottom 0: 25.41,175.72 25.02,175.51
S$1977
  Bottom 0: 25.02,175.51 24.67,175.22
S$1978
  Bottom 0: 24.67,175.22 24.39,174.88
S$1979
  Bottom 0: 24.39,174.88 24.18,174.48
S$1980
  Bottom 0: 24.18,174.48 24.05,174.06
S$1981
  Bottom 0: 24.05,174.06 24,173.61
S$1982
  Bottom 0: 24,173.61 24.05,173.16
S$1983
  Bottom 0: 24.05,173.16 24.18,172.74
S$1984
  Bottom 0: 24.18,172.74 24.39,172.34
S$1985
  Bottom 0: 24.39,172.34 24.67,171.99
S$1986
  Bottom 0: 24.67,171.99 25.02,171.71
S$1987
  Bottom 0: 25.02,171.71 25.39,171.51
S$1988
  Bottom 0: 25.39,171.51 24.07,171.51
S$1989
  Bottom 0: 24.07,171.51 24,171.51
S$1990
  Bottom 0: 24,171.51 23.93,171.49
S$1991
  Bottom 0: 23.93,171.49 23.87,171.47
S$1992
  Bottom 0: 23.87,171.47 23.81,171.43
S$1993
  Bottom 0: 23.81,171.43 23.75,171.38
S$1994
  Bottom 0: 23.75,171.38 21.93,169.56
S$1995
  Bottom 0: 21.93,169.56 21.93,170.39
S$1996
  Bottom 0: 21.93,170.39 22,170.46
S$1997
  Bottom 0: 22,170.46 22.04,170.46
S$1998
  Bottom 0: 22.04,170.46 22.18,170.48
S$1999
  Bottom 0: 22.18,170.48 22.3,170.55
S$2000
  Bottom 0: 22.3,170.55 22.4,170.64
S$2001
  Bottom 0: 22.4,170.64 22.46,170.76
S$2002
  Bottom 0: 22.46,170.76 22.48,170.9
S$2003
  Bottom 0: 22.48,170.9 22.48,174.25
S$2004
  Bottom 0: 22.48,174.25 25.33,177.1
S$2005
  Bottom 0: 25.33,177.1 25.37,177.17
S$2006
  Bottom 0: 25.37,177.17 25.4,177.2
S$2007
  Bottom 0: 25.4,177.2 25.41,177.24
S$2008
  Bottom 0: 25.41,177.24 25.45,177.3
S$2009
  Bottom 0: 25.45,177.3 25.45,177.36
S$2010
  Bottom 0: 25.45,177.36 25.46,177.42
S$2011
  Bottom 0: 25.46,177.42 25.46,177.55
S$2012
  Bottom 0: 25.46,177.55 25.91,177.55
S$2013
  Bottom 0: 25.91,177.55 25.98,177.56
S$2014
  Bottom 0: 25.98,177.56 26.05,177.6
S$2015
  Bottom 0: 26.05,177.6 26.11,177.65
S$2016
  Bottom 0: 26.11,177.65 26.15,177.72
S$2017
  Bottom 0: 26.15,177.72 26.16,177.8
S$2018
  Bottom 0: 26.16,177.8 26.16,179.58
S$2019
  Bottom 0: 26.16,179.58 26.15,179.65
S$2020
  Bottom 0: 26.15,179.65 26.11,179.72
S$2021
  Bottom 0: 26.11,179.72 26.05,179.78
S$2022
  Bottom 0: 26.05,179.78 25.98,179.82
S$2023
  Bottom 0: 25.98,179.82 25.91,179.83
S$2024
  Bottom 0: 25.91,179.83 24.13,179.83
S$2025
  Bottom 0: 24.13,179.83 24.05,179.82
S$2026
  Bottom 0: 24.05,179.82 23.98,179.78
S$2027
  Bottom 0: 23.98,179.78 23.92,179.72
S$2028
  Bottom 0: 23.92,179.72 23.89,179.65
S$2029
  Bottom 0: 23.89,179.65 23.88,179.58
S$2030
  Bottom 0: 23.88,179.58 23.88,177.8
S$2031
  Bottom 0: 23.88,177.8 23.89,177.72
S$2032
  Bottom 0: 23.89,177.72 23.92,177.65
S$2033
  Bottom 0: 23.92,177.65 23.98,177.6
S$2034
  Bottom 0: 23.98,177.6 24.05,177.56
S$2035
  Bottom 0: 24.05,177.56 24.13,177.55
S$2036
  Bottom 0: 24.13,177.55 24.51,177.55
S$2037
  Bottom 0: 24.51,177.55 21.73,174.76
S$2038
  Bottom 0: 21.73,174.76 21.69,174.7
S$2039
  Bottom 0: 21.69,174.7 21.65,174.64
S$2040
  Bottom 0: 21.65,174.64 21.62,174.58
S$2041
  Bottom 0: 21.62,174.58 21.61,174.51
S$2042
  Bottom 0: 21.61,174.51 21.6,174.44
S$2043
  Bottom 0: 21.6,174.44 21.6,171.29
S$2044
  Bottom 0: 21.6,171.29 21.55,171.26
S$2045
  Bottom 0: 21.55,171.26 21.5,171.22
S$2046
  Bottom 0: 21.5,171.22 21.17,170.89
S$2047
  Bottom 0: 21.17,170.89 21.13,170.84
S$2048
  Bottom 0: 21.13,170.84 21.09,170.78
S$2049
  Bottom 0: 21.09,170.78 21.06,170.71
S$2050
  Bottom 0: 21.06,170.71 21.05,170.65
S$2051
  Bottom 0: 21.05,170.65 21.04,170.58
S$2052
  Bottom 0: 21.04,170.58 21.04,166.64
S$2053
  Bottom 0: 21.04,166.64 21.05,166.57
S$2054
  Bottom 0: 21.05,166.57 21.06,166.5
S$2055
  Bottom 0: 21.06,166.5 21.09,166.44
S$2056
  Bottom 0: 21.09,166.44 21.13,166.38
S$2057
  Bottom 0: 21.13,166.38 21.17,166.32
S$2058
  Bottom 0: 21.17,166.32 21.52,165.97
S$2059
  Bottom 0: 21.52,165.97 21.38,165.75
S$2060
  Bottom 0: 21.38,165.75 21.29,165.43
S$2061
  Bottom 0: 21.29,165.43 21.29,165.11
S$2062
  Bottom 0: 21.29,165.11 21.38,164.79
S$2063
  Bottom 0: 21.38,164.79 21.55,164.52
S$2064
  Bottom 0: 21.55,164.52 21.79,164.3
S$2065
  Bottom 0: 21.79,164.3 22.08,164.15
S$2066
  Bottom 0: 22.08,164.15 22.4,164.08
S$2067
  Bottom 0: 22.4,164.08 22.72,164.1
S$2068
  Bottom 0: 22.72,164.1 23.03,164.21
S$2069
  Bottom 0: 23.03,164.21 23.29,164.4
S$2070
  Bottom 0: 23.29,164.4 23.5,164.65
S$2071
  Bottom 0: 23.5,164.65 23.62,164.95
S$2072
  Bottom 0: 23.62,164.95 23.67,165.27
S$2073
  Bottom 0: 23.67,165.27 23.62,165.59
S$2074
  Bottom 0: 23.62,165.59 23.58,165.7
S$2075
  Bottom 0: 23.58,165.7 24.38,164.9
S$2076
  Bottom 0: 24.38,164.9 24.38,158.33
S$2077
  Bottom 0: 24.38,158.33 24.38,158.25
S$2078
  Bottom 0: 24.38,158.25 24.4,158.19
S$2079
  Bottom 0: 24.4,158.19 24.43,158.13
S$2080
  Bottom 0: 24.43,158.13 24.46,158.07
S$2081
  Bottom 0: 24.46,158.07 24.51,158.02
S$2082
  Bottom 0: 24.51,158.02 29.34,153.18
S$2083
  Bottom 0: 29.34,153.18 29.4,153.14
S$2084
  Bottom 0: 29.4,153.14 23.18,153.14
S$2085
  Bottom 0: 23.18,153.14 23.18,159.38
S$2086
  Bottom 0: 23.18,159.38 23.17,159.46
S$2087
  Bottom 0: 23.17,159.46 23.16,159.52
S$2088
  Bottom 0: 23.16,159.52 23.13,159.58
S$2089
  Bottom 0: 23.13,159.58 23.09,159.64
S$2090
  Bottom 0: 23.09,159.64 23.05,159.7
S$2091
  Bottom 0: 23.05,159.7 12.29,170.45
S$2092
  Bottom 0: 12.29,170.45 12.4,170.72
S$2093
  Bottom 0: 12.4,170.72 12.45,171.07
S$2094
  Bottom 0: 12.45,171.07 12.4,171.41
S$2095
  Bottom 0: 12.4,171.41 12.27,171.74
S$2096
  Bottom 0: 12.27,171.74 12.06,172.02
S$2097
  Bottom 0: 12.06,172.02 11.8,172.25
S$2098
  Bottom 0: 11.8,172.25 11.48,172.4
S$2099
  Bottom 0: 11.48,172.4 11.13,172.46
S$2100
  Bottom 0: 11.13,172.46 10.78,172.44
S$2101
  Bottom 0: 10.78,172.44 10.46,172.33
S$2102
  Bottom 0: 10.46,172.33 10.16,172.15
S$2103
  Bottom 0: 10.16,172.15 9.97,171.95
S$2104
  Bottom 0: 9.97,171.95 9.97,171.97
S$2105
  Bottom 0: 9.97,171.97 10.17,172.16
S$2106
  Bottom 0: 10.17,172.16 10.23,172.23
S$2107
  Bottom 0: 10.23,172.23 10.27,172.3
S$2108
  Bottom 0: 10.27,172.3 10.31,172.38
S$2109
  Bottom 0: 10.31,172.38 10.33,172.47
S$2110
  Bottom 0: 10.33,172.47 10.34,172.56
S$2111
  Bottom 0: 10.34,172.56 10.34,177.43
S$2112
  Bottom 0: 10.34,177.43 10.33,177.52
S$2113
  Bottom 0: 10.33,177.52 10.31,177.61
S$2114
  Bottom 0: 10.31,177.61 10.27,177.69
S$2115
  Bottom 0: 10.27,177.69 10.23,177.76
S$2116
  Bottom 0: 10.23,177.76 10.17,177.83
S$2117
  Bottom 0: 10.17,177.83 9.61,178.39
S$2118
  Bottom 0: 9.61,178.39 9.65,178.69
S$2119
  Bottom 0: 9.65,178.69 9.6,179.01
S$2120
  Bottom 0: 9.6,179.01 9.47,179.31
S$2121
  Bottom 0: 9.47,179.31 9.26,179.55
S$2122
  Bottom 0: 9.26,179.55 8.98,179.73
S$2123
  Bottom 0: 8.98,179.73 8.67,179.82
S$2124
  Bottom 0: 8.67,179.82 8.35,179.82
S$2125
  Bottom 0: 8.35,179.82 8.03,179.73
S$2126
  Bottom 0: 8.03,179.73 7.76,179.55
S$2127
  Bottom 0: 7.76,179.55 7.55,179.31
S$2128
  Bottom 0: 7.55,179.31 7.41,179.01
S$2129
  Bottom 0: 7.41,179.01 7.37,178.69
S$2130
  Bottom 0: 7.37,178.69 7.41,178.37
S$2131
  Bottom 0: 7.41,178.37 7.55,178.07
S$2132
  Bottom 0: 7.55,178.07 7.76,177.82
S$2133
  Bottom 0: 7.76,177.82 8.03,177.65
S$2134
  Bottom 0: 8.03,177.65 8.35,177.56
S$2135
  Bottom 0: 8.35,177.56 8.67,177.56
S$2136
  Bottom 0: 8.67,177.56 8.8,177.6
S$2137
  Bottom 0: 8.8,177.6 9.2,177.19
S$2138
  Bottom 0: 9.2,177.19 9.2,174.77
S$2139
  Bottom 0: 9.2,174.77 9.14,174.88
S$2140
  Bottom 0: 9.14,174.88 8.85,175.22
S$2141
  Bottom 0: 8.85,175.22 8.51,175.51
S$2142
  Bottom 0: 8.51,175.51 8.11,175.72
S$2143
  Bottom 0: 8.11,175.72 7.68,175.85
S$2144
  Bottom 0: 7.68,175.85 7.24,175.9
S$2145
  Bottom 0: 7.24,175.9 6.79,175.85
S$2146
  Bottom 0: 6.79,175.85 6.37,175.72
S$2147
  Bottom 0: 6.37,175.72 5.97,175.51
S$2148
  Bottom 0: 5.97,175.51 5.62,175.22
S$2149
  Bottom 0: 5.62,175.22 5.34,174.88
S$2150
  Bottom 0: 5.34,174.88 5.13,174.48
S$2151
  Bottom 0: 5.13,174.48 5,174.06
S$2152
  Bottom 0: 5,174.06 4.95,173.61
S$2153
  Bottom 0: 4.95,173.61 5,173.16
S$2154
  Bottom 0: 5,173.16 5.13,172.74
S$2155
  Bottom 0: 5.13,172.74 5.34,172.34
S$2156
  Bottom 0: 5.34,172.34 5.62,171.99
S$2157
  Bottom 0: 5.62,171.99 5.97,171.71
S$2158
  Bottom 0: 5.97,171.71 6.37,171.5
S$2159
  Bottom 0: 6.37,171.5 6.79,171.37
S$2160
  Bottom 0: 6.79,171.37 7.24,171.32
S$2161
  Bottom 0: 7.24,171.32 7.68,171.37
S$2162
  Bottom 0: 7.68,171.37 8.11,171.5
S$2163
  Bottom 0: 8.11,171.5 8.51,171.71
S$2164
  Bottom 0: 8.51,171.71 8.84,171.98
S$2165
  Bottom 0: 8.84,171.98 8.84,164.17
S$2166
  Bottom 0: 8.84,164.17 8.84,164.08
S$2167
  Bottom 0: 8.84,164.08 8.86,163.99
S$2168
  Bottom 0: 8.86,163.99 8.9,163.91
S$2169
  Bottom 0: 8.9,163.91 8.95,163.84
S$2170
  Bottom 0: 8.95,163.84 9,163.77
S$2171
  Bottom 0: 9,163.77 12.4,160.37
S$2172
  Bottom 0: 12.4,160.37 12.31,160.26
S$2173
  Bottom 0: 12.31,160.26 12.17,159.96
S$2174
  Bottom 0: 12.17,159.96 12.13,159.64
S$2175
  Bottom 0: 12.13,159.64 12.17,159.32
S$2176
  Bottom 0: 12.17,159.32 12.31,159.02
S$2177
  Bottom 0: 12.31,159.02 12.52,158.78
S$2178
  Bottom 0: 12.52,158.78 12.8,158.6
S$2179
  Bottom 0: 12.8,158.6 13.11,158.51
S$2180
  Bottom 0: 13.11,158.51 13.43,158.51
S$2181
  Bottom 0: 13.43,158.51 13.74,158.6
S$2182
  Bottom 0: 13.74,158.6 14.02,158.78
S$2183
  Bottom 0: 14.02,158.78 14.23,159.02
S$2184
  Bottom 0: 14.23,159.02 14.37,159.32
S$2185
  Bottom 0: 14.37,159.32 14.41,159.64
S$2186
  Bottom 0: 14.41,159.64 14.37,159.96
S$2187
  Bottom 0: 14.37,159.96 14.23,160.26
S$2188
  Bottom 0: 14.23,160.26 14.02,160.5
S$2189
  Bottom 0: 14.02,160.5 13.74,160.68
S$2190
  Bottom 0: 13.74,160.68 13.67,160.7
S$2191
  Bottom 0: 13.67,160.7 13.67,160.71
S$2192
  Bottom 0: 13.67,160.71 9.97,164.4
S$2193
  Bottom 0: 9.97,164.4 9.97,164.75
S$2194
  Bottom 0: 9.97,164.75 10.12,164.52
S$2195
  Bottom 0: 10.12,164.52 10.36,164.29
S$2196
  Bottom 0: 10.36,164.29 10.65,164.15
S$2197
  Bottom 0: 10.65,164.15 10.97,164.08
S$2198
  Bottom 0: 10.97,164.08 11.29,164.1
S$2199
  Bottom 0: 11.29,164.1 11.38,164.13
S$2200
  Bottom 0: 11.38,164.13 13.02,162.49
S$2201
  Bottom 0: 13.02,162.49 13.08,162.43
S$2202
  Bottom 0: 13.08,162.43 13.16,162.38
S$2203
  Bottom 0: 13.16,162.38 13.24,162.35
S$2204
  Bottom 0: 13.24,162.35 13.33,162.33
S$2205
  Bottom 0: 13.33,162.33 13.42,162.33
S$2206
